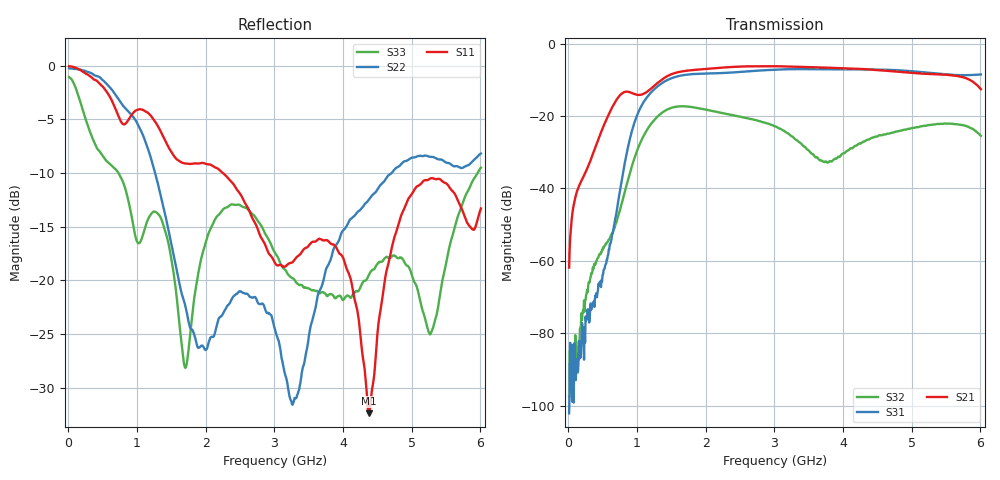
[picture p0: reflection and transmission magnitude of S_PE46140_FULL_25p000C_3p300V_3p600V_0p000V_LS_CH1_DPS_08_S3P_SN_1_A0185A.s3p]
! Device ID: PE46140_FULL
! File Path: z:\PE46140\MajorStates\25p000C\3p300\LS_CH1_DPS_08\PE46140_FULL_25p000C_3p300V_3p600V_0p000V_LS_CH1_DPS_08_S3P_SN_1_A0185A.s3p
! Serial: 1
! Lot: A0185A
! Temp: 25.000C
! VDD: 3.300
! VSS: 0.000
! Control_Hi: 3.600
! Control_Lo: 0.000
! Logic State: LS_CH1_DPS_08
! Port 1: RFIN
! Port 2: RFOUT1
! Port 3: RFOUT2
! ThroughPath:1-2
! IDD: 0.0003110989
! ISS: -2.092e-007
! Comment:
#  Hz  S  RI  R  50
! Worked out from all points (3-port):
!   801 points, 10 MHz to 6.01 GHz, reference 50 ohm
!   strongest paths, dB at 10 MHz, 1.51 GHz, 3.01 GHz, 4.51 GHz, 6.01 GHz:
!     S21: -61.8, -8.4, -6.2, -7.3, -12.6
!     S31: -102.1, -9.5, -7.2, -7.2, -8.5
!     S32: -97.6, -17.7, -22.9, -25.5, -25.4
!   lowest |S11| = -32.4 dB at 4.375 GHz (marker M1), VSWR 1.05, Z = 52.4 + j0.34 ohm
!   |S11| at or under -10 dB: 2.251 GHz to end of sweep
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1e7  0.9924 -0.0706  0.00019 0.000797  -1.75e-05 8.15e-07
     0.000278 0.000761  0.9732 -0.0266  -1.83e-05 4.1e-05
     2.68e-06 7.39e-06  -1.15e-05 6.56e-06  0.8809 -0.083
3.55e8  -0.395 -0.7766  -0.00349 0.0296  -2.98e-05 0.000216
        -0.00358 0.0296  0.6238 -0.668  -0.000612 0.000363
        1.14e-06 0.000259  -0.000665 0.000457  -0.4042 -0.2106
1.15e9  -0.5511 0.2532  0.2067 -0.069  -0.1734 -0.063
        0.2073 -0.0688  -0.4062 -0.0957  -0.0611 -0.0238
        -0.1737 -0.0633  -0.0611 -0.0237  0.1533 0.1115
1.705e9  -0.2398 0.2556  -0.0571 -0.4171  0.2715 0.2524
         -0.0572 -0.4172  -0.019 0.0733  0.1305 -0.0377
         0.2717 0.2529  0.1307 -0.0375  -0.039 -0.00389
1.9675e9  -0.1835 0.3007  -0.3102 -0.3189  0.383 -0.0478
          -0.31 -0.3191  -0.00129 0.049  -0.00667 -0.1244
          0.3832 -0.0477  -0.0064 -0.1244  0.0428 0.1317
3.01e9  0.0116 0.1199  -0.0481 0.4848  -0.3798 -0.2173
        -0.049 0.4851  0.059 0.00432  0.0587 0.0414
        -0.3802 -0.2175  0.0589 0.0413  0.1253 -0.049
3.985e9  -0.00967 0.1301  0.437 -0.1386  -0.0518 0.439
         0.4373 -0.1383  0.099 0.136  -0.00556 0.0295
         -0.0511 0.4385  -0.00551 0.0295  0.0799 -0.0197
4.375e9  0.0239 0.00324  0.1987 -0.3931  0.2577 0.3552
         0.1996 -0.3932  0.1999 0.1276  0.0472 -0.00176
         0.2581 0.3551  0.0474 -0.00198  0.1009 -0.0309
4.96e9  -0.136 -0.2001  -0.2583 -0.3008  0.4131 -0.0704
        -0.2581 -0.3016  0.366 -0.00719  -0.0467 -0.0474
        0.4139 -0.0701  -0.047 -0.0474  0.0874 -0.0753
6.01e9  -0.1319 -0.1715  0.0244 0.2333  -0.1525 -0.3415
        0.0244 0.2339  0.2264 -0.3174  0.0475 0.0242
        -0.1539 -0.3422  0.0476 0.0241  0.3141 0.1171
